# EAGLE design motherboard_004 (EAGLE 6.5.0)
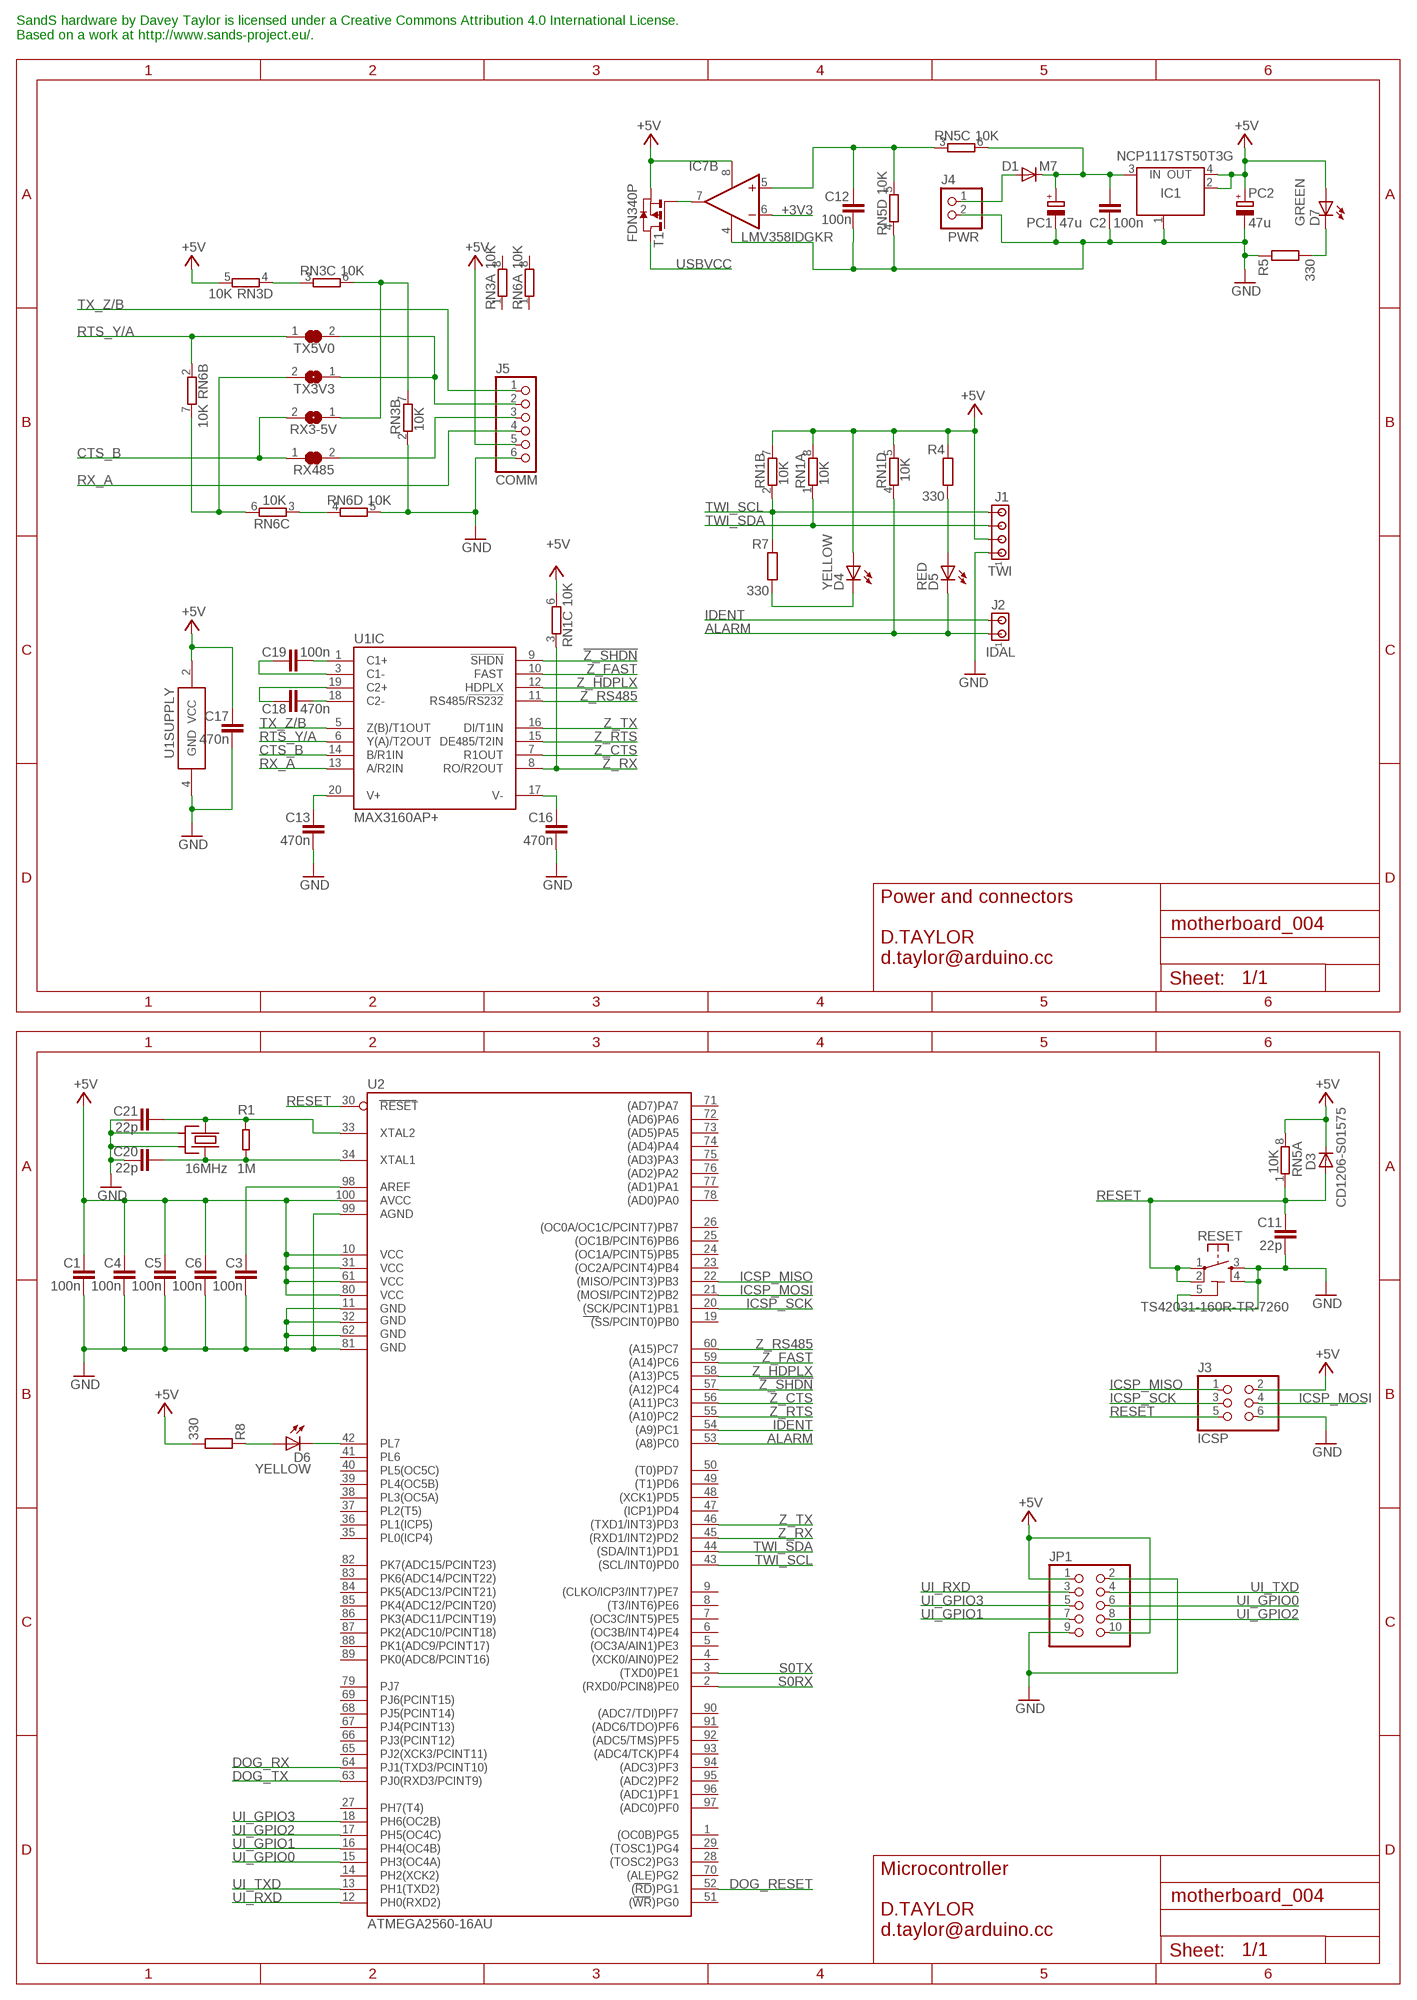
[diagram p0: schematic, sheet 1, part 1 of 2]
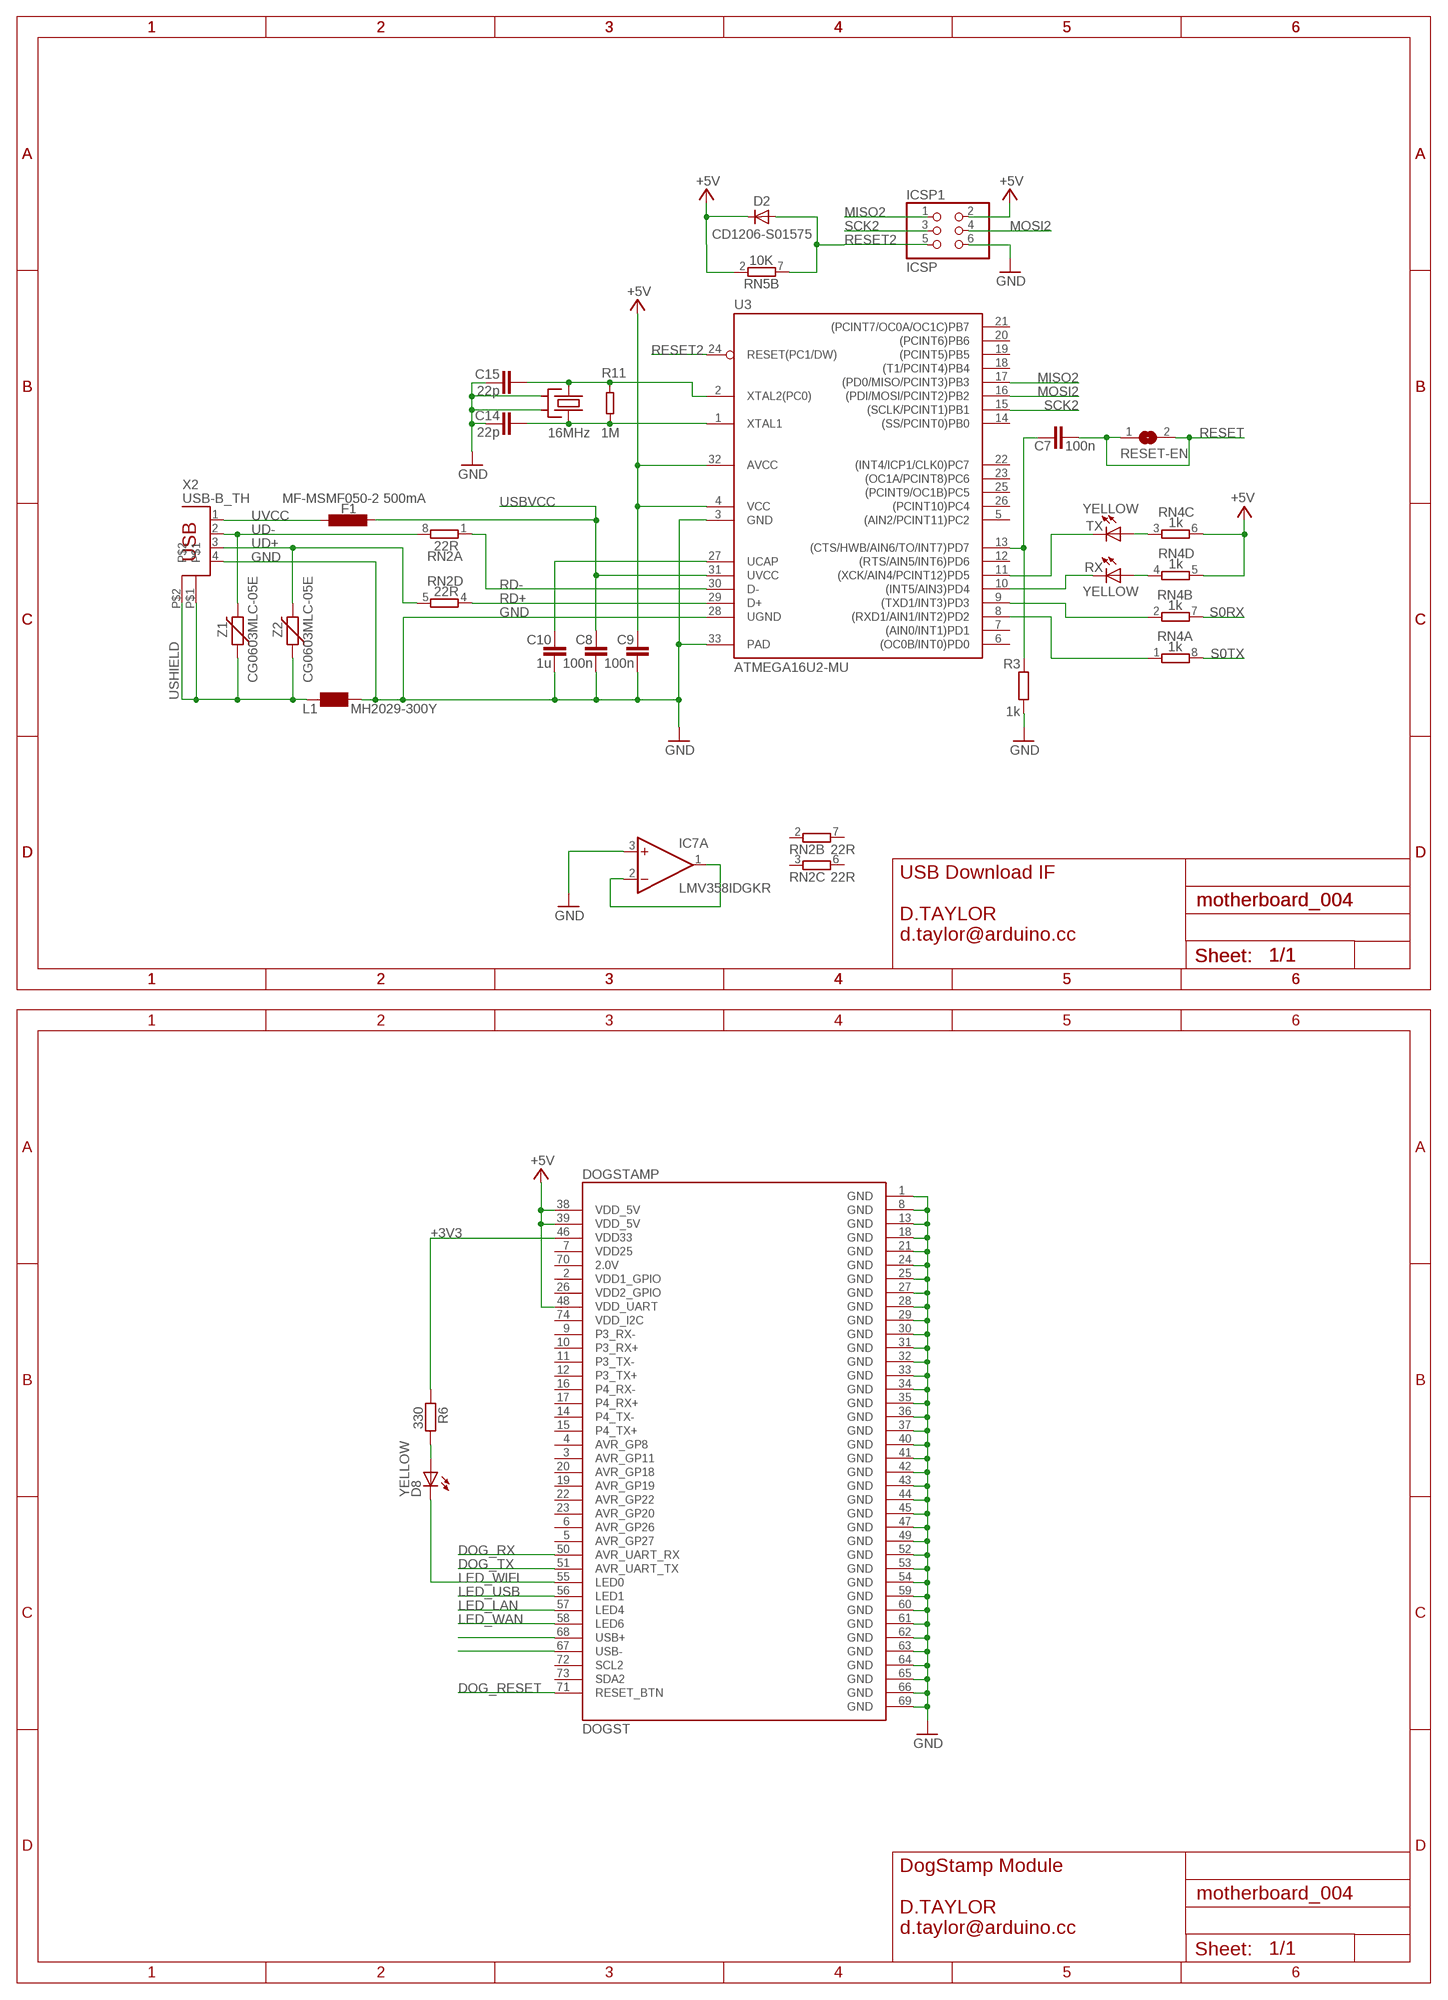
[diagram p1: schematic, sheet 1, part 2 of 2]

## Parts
C1  100n  C-EU0603-RND  [C0603-ROUND]
C2  100n  C-EU0603-RND  [C0603-ROUND]
C3  100n  C-EU0603-RND  [C0603-ROUND]
C4  100n  C-EU0603-RND  [C0603-ROUND]
C5  100n  C-EU0603-RND  [C0603-ROUND]
C6  100n  C-EU0603-RND  [C0603-ROUND]
C7  100n  C-EU0603-RND  [C0603-ROUND]
C8  100n  C-EU0603-RND  [C0603-ROUND]
C9  100n  C-EU0603-RND  [C0603-ROUND]
C10  1u  C-EU0603-RND  [C0603-ROUND]
C11  22p  C-EU0603-RND  [C0603-ROUND]
C12  100n  C-EU0603-RND  [C0603-ROUND]
C13  470n  C-EU0603-RND  [C0603-ROUND]
C14  22p  C-EU0603-RND  [C0603-ROUND]
C15  22p  C-EU0603-RND  [C0603-ROUND]
C16  470n  C-EU0603-RND  [C0603-ROUND]
C17  470n  C-EU0603-RND  [C0603-ROUND]
C18  470n  C-EU0603-RND  [C0603-ROUND]
C19  100n  C-EU0603-RND  [C0603-ROUND]
C20  22p  C-EU0603-RND  [C0603-ROUND]
C21  22p  C-EU0603-RND  [C0603-ROUND]
D1  M7  DIODE-SMB  [SMB]
D2  CD1206-S01575  DIODE-MINIMELF  [MINIMELF]
D3  CD1206-S01575  DIODE-MINIMELF  [MINIMELF]
D4  YELLOW  LEDCHIP-LED0805  [CHIP-LED0805]
D5  RED  LEDCHIP-LED0805  [CHIP-LED0805]
D6  YELLOW  LEDCHIP-LED0805  [CHIP-LED0805]
D7  GREEN  LEDCHIP-LED0805  [CHIP-LED0805]
D8  YELLOW  LEDCHIP-LED0805  [CHIP-LED0805]
DOGSTAMP  DOGST  [DOGST]
F1  MF-MSMF050-2 500mA  L-EUL1812  [L1812]
IC1  NCP1117ST50T3G  MC33269ST-3.3T3  [SOT223]
IC7  LMV358IDGKR  LMV358MMX  [MSOP08]
ICSP1  ICSP  PINHD-2X3  [2X03]
J1  TWI  MTA04-100  [10X04MTA]
J2  IDAL  MTA02-100  [10X02MTA]
J3  ICSP  PINHD-2X3  [2X03]
J4  PWR  MKDS_1,5/2-5,08  [MKDS1,5/2-5,08]
J5  COMM  PINHD-1X6  [1X06]
JP1  PINHD-2X5  [2X05]
L1  MH2029-300Y  WE-CBF_0805  [0805]
PC1  47u  CPOL-EUD  [PANASONIC_D]
PC2  47u  CPOL-EUD  [PANASONIC_D]
R1  1M  R-EU_0603-RND  [R0603-ROUND]
R3  1k  R-EU_R0603  [R0603-ROUND]
R4  330  R-EU_R0603  [R0603-ROUND]
R5  330  R-EU_R0603  [R0603-ROUND]
R6  330  R-EU_R0603  [R0603-ROUND]
R7  330  R-EU_R0603  [R0603-ROUND]
R8  330  R-EU_R0603  [R0603-ROUND]
R11  1M  R-EU_0603-RND  [R0603-ROUND]
RESET  TS42031-160R-TR-7260  TS42  [TS42]
RESET-EN  SJ  [SJ]
RN1  10K  4R-NCAT16  [CAT16]
RN2  22R  4R-NCAY16  [CAY16]
RN3  10K  4R-NCAT16  [CAT16]
RN4  1k  4R-NCAY16  [CAY16]
RN5  10K  4R-NCAT16  [CAT16]
RN6  10K  4R-NCAT16  [CAT16]
RX  YELLOW  LEDCHIP-LED0805  [CHIP-LED0805]
RX3-5V  SJ-NO  [SJ]
RX485  SJ-NC  [SJ-NC]
T1  FDN340P  PMOSSOT23  [SOT-23]
TX  YELLOW  LEDCHIP-LED0805  [CHIP-LED0805]
TX3V3  SJ-NO  [SJ]
TX5V0  SJ-NC  [SJ-NC]
U1  MAX3160AP+  [SSOP20]
U2  ATMEGA2560-16AU  ATMEGA25602560-16AU  [TQFP100]
U3  ATMEGA16U2-MU  [MLF32]
X1  16MHz  CRYSTAL2-KX7  [XTAL-3.2-2.5]
X2  USB-B_TH  PN61729  [PN61729]
X3  16MHz  CRYSTAL2-KX7  [XTAL-3.2-2.5]
Z1  CG0603MLC-05E  VARISTORCN0603  [CT/CN0603]
Z2  CG0603MLC-05E  VARISTORCN0603  [CT/CN0603]

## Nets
!Z_SHDN!: U1.9(IC:!SHDN!) U2.57((A12)PC4)
+3V3 [power]: DOGSTAMP.46(VDD33) IC7.6(B:-IN) R6.2
+5V: C1.1 C4.1 C5.1 C6.1 C9.1 C17.1 D2.C D3.C D4.A D7.A DOGSTAMP.38(VDD_5V) DOGSTAMP.39(VDD_5V) DOGSTAMP.48(VDD_UART) IC1.2(OUT) IC1.4(OUT) IC7.8(P:V+) ICSP1.2 J1.2 J3.2 J5.5 JP1.1 JP1.10 PC2.+ R4.2 R8.1 RN1.5 RN1.6 RN1.7 RN1.8 RN3.5 RN4.5 RN4.6 RN5.2 RN5.8 T1.2(S) U1.2(SUPPLY:VCC) U2.10(VCC) U2.31(VCC1) U2.61(VCC2) U2.80(VCC3) U2.100(AVCC) U3.4(VCC) U3.32(AVCC)
ALARM: D5.C J2.1 RN1.4 U2.53((A8)PC0)
CMP: C12.2 IC7.5(B:+IN) RN5.3 RN5.5
CTS_B: RX3-5V.2 RX485.1 U1.14(IC:B/R1IN)
DOG_RESET: DOGSTAMP.71(RESET_BTN) U2.52((RD)PG1)
DOG_RX: DOGSTAMP.50(AVR_UART_RX) U2.64(PJ1(TXD3/PCINT10))
DOG_TX: DOGSTAMP.51(AVR_UART_TX) U2.63(PJ0(RXD3/PCINT9))
DTR: C7.1 R3.2 U3.13((CTS/HWB/AIN6/TO/INT7)PD7)
GATE_CMD: IC7.7(B:OUT) T1.3(G)
GND: C1.2 C2.2 C3.2 C4.2 C5.2 C6.2 C8.2 C9.2 C10.2 C11.2 C12.1 C13.2 C14.2 C15.2 C16.2 C17.2 C20.2 C21.2 DOGSTAMP.1(GND) DOGSTAMP.8(GND) DOGSTAMP.13(GND) DOGSTAMP.18(GND) DOGSTAMP.21(GND) DOGSTAMP.24(GND) DOGSTAMP.25(GND) DOGSTAMP.27(GND) DOGSTAMP.28(GND) DOGSTAMP.29(GND) DOGSTAMP.30(GND) DOGSTAMP.31(GND) DOGSTAMP.32(GND) DOGSTAMP.33(GND) DOGSTAMP.34(GND) DOGSTAMP.35(GND) DOGSTAMP.36(GND) DOGSTAMP.37(GND) DOGSTAMP.40(GND) DOGSTAMP.41(GND) DOGSTAMP.42(GND) DOGSTAMP.43(GND) DOGSTAMP.44(GND) DOGSTAMP.45(GND) DOGSTAMP.47(GND) DOGSTAMP.49(GND) DOGSTAMP.52(GND) DOGSTAMP.53(GND) DOGSTAMP.54(GND) DOGSTAMP.59(GND) DOGSTAMP.60(GND) DOGSTAMP.61(GND) DOGSTAMP.62(GND) DOGSTAMP.63(GND) DOGSTAMP.64(GND) DOGSTAMP.65(GND) DOGSTAMP.66(GND) DOGSTAMP.69(GND) IC1.1(GND/ADJ) IC7.3(A:+IN) IC7.4(P:V-) ICSP1.6 J1.1 J3.6 J4.2 J5.6 JP1.2 JP1.9 L1.1 PC1.- PC2.- R3.1 R5.2 RESET.3 RESET.4 RESET.5(5-GND) RN3.2 RN5.4 RN6.5 U1.4(SUPPLY:GND) U2.11(GND) U2.32(GND1) U2.62(GND2) U2.81(GND3) U2.99(AGND) U3.3(GND) U3.28(UGND) U3.33(PAD) X1.2(SH1) X1.4(SH2) X2.4 X3.2(SH1) X3.4(SH2)
ICSP_MISO: J3.1 U2.22((MISO/PCINT3)PB3)
ICSP_MOSI: J3.4 U2.21((MOSI/PCINT2)PB2)
ICSP_SCK: J3.3 U2.20((SCK/PCINT1)PB1)
IDENT: J2.2 U2.54((A9)PC1)
LED_LAN: DOGSTAMP.57(LED4)
LED_USB: DOGSTAMP.56(LED1)
LED_WAN: DOGSTAMP.58(LED6)
LED_WIFI: D8.C DOGSTAMP.55(LED0)
M8RXD: RN4.2 U3.9((TXD1/INT3)PD3)
M8TXD: RN4.1 U3.8((RXD1/AIN1/INT2)PD2)
MISO2: ICSP1.1 U3.17((PD0/MISO/PCINT3)PB3)
MOSI2: ICSP1.4 U3.16((PDI/MOSI/PCINT2)PB2)
N$1: C3.1 U2.98(AREF)
N$2: IC7.1(A:OUT) IC7.2(A:-IN)
N$3: C14.1 R11.1 U3.1(XTAL1) X1.3(X2)
N$4: DOGSTAMP.68(USB+)
N$5: D5.A R4.1
N$6: C19.2 U1.1(IC:C1+)
N$7: C18.2 U1.18(IC:C2-)
N$8: C18.1 U1.19(IC:C2+)
N$9: C19.1 U1.3(IC:C1-)
N$10: C13.1 U1.20(IC:V+)
N$11: C16.1 U1.17(IC:V-)
N$12: D7.C R5.1
N$13: D8.A R6.1
N$14: D4.C R7.1
N$15: D6.C U2.42(PL7)
N$16: D6.A R8.2
N$17: DOGSTAMP.67(USB-)
N$18: RN3.3 RN3.4
N$19 [power]: RN3.6 RN3.7 RX3-5V.1
N$20: J5.3 RX485.2
N$21: C20.1 R1.1 U2.34(XTAL1) X3.3(X2)
N$22: J5.2 TX3V3.1 TX5V0.2
N$23: RN6.6 RN6.7 TX3V3.2
N$24: RN6.3 RN6.4
N$54: RN4.4 RX.A
N$55: RN4.3 TX.A
PWRIN [power]: D1.A J4.1
RD+: RN2.4 U3.29(D+)
RD-: RN2.1 U3.30(D-)
RESET: C7.2 C11.1 D3.A J3.5 RESET-EN.1 RESET-EN.2 RESET.1 RESET.2 RN5.1 U2.30(RESET)
RESET2: D2.A ICSP1.5 RN5.7 U3.24(RESET(PC1/DW))
RTS_Y/A: RN6.2 TX5V0.1 U1.6(IC:Y(A)/T2OUT)
RX_A: J5.4 U1.13(IC:A/R2IN)
RXL: RX.C U3.10((INT5/AIN3)PD4)
S0RX: RN4.7 U2.2((RXD0/PCIN8)PE0)
S0TX: RN4.8 U2.3((TXD0)PE1)
SCK2: ICSP1.3 U3.15((SCLK/PCINT1)PB1)
TWI_SCL: J1.4 R7.2 RN1.2 U2.43((SCL/INT0)PD0)
TWI_SDA: J1.3 RN1.1 U2.44((SDA/INT1)PD1)
TX_Z/B: J5.1 U1.5(IC:Z(B)/T1OUT)
TXL: TX.C U3.11((XCK/AIN4/PCINT12)PD5)
UD+: RN2.5 X2.3 Z2.2
UD-: RN2.8 X2.2 Z1.2
UI_GPIO0: JP1.6 U2.15(PH3(OC4A))
UI_GPIO1: JP1.7 U2.16(PH4(OC4B))
UI_GPIO2: JP1.8 U2.17(PH5(OC4C))
UI_GPIO3: JP1.5 U2.18(PH6(OC2B))
UI_RXD: JP1.3 U2.12(PH0(RXD2))
UI_TXD: JP1.4 U2.13(PH1(TXD2))
USBVCC [power usb]: C8.1 F1.1 T1.1(D) U3.31(UVCC)
USHIELD [gnd]: L1.2 X2.P$1 X2.P$2 Z1.1 Z2.1
UVCC [power usb]: F1.2 X2.1
VIN [power]: C2.1 D1.C IC1.3(IN) PC1.+ RN5.6
VUCAP: C10.1 U3.27(UCAP)
XT1: C21.1 R1.2 U2.33(XTAL2) X3.1(X1)
XT2: C15.1 R11.2 U3.2(XTAL2(PC0)) X1.1(X1)
Z_CTS: U1.7(IC:R1OUT) U2.56((A11)PC3)
Z_FAST: U1.10(IC:FAST) U2.59((A14)PC6)
Z_HDPLX: U1.12(IC:HDPLX) U2.58((A13)PC5)
Z_RS485: U1.11(IC:RS485/!RS232!) U2.60((A15)PC7)
Z_RTS: U1.15(IC:DE485/T2IN) U2.55((A10)PC2)
Z_RX: RN1.3 U1.8(IC:RO/R2OUT) U2.45((RXD1/INT2)PD2)
Z_TX: U1.16(IC:DI/T1IN) U2.46((TXD1/INT3)PD3)
Unconnected: DOGSTAMP.2(VDD1_GPIO) DOGSTAMP.3(AVR_GP11) DOGSTAMP.4(AVR_GP8) DOGSTAMP.5(AVR_GP27) DOGSTAMP.6(AVR_GP26) DOGSTAMP.7(VDD25) DOGSTAMP.9(P3_RX-) DOGSTAMP.10(P3_RX+) DOGSTAMP.11(P3_TX-) DOGSTAMP.12(P3_TX+) DOGSTAMP.14(P4_TX-) DOGSTAMP.15(P4_TX+) DOGSTAMP.16(P4_RX-) DOGSTAMP.17(P4_RX+) DOGSTAMP.19(AVR_GP19) DOGSTAMP.20(AVR_GP18) DOGSTAMP.22(AVR_GP22) DOGSTAMP.23(AVR_GP20) DOGSTAMP.26(VDD2_GPIO) DOGSTAMP.70(2.0V) DOGSTAMP.72(SCL2) DOGSTAMP.73(SDA2) DOGSTAMP.74(VDD_I2C) RN2.2 RN2.3 RN2.6 RN2.7 RN3.1 RN3.8 RN6.1 RN6.8 U2.1((OC0B)PG5) U2.4((XCK0/AIN0)PE2) U2.5((OC3A/AIN1)PE3) U2.6((OC3B/INT4)PE4) U2.7((OC3C/INT5)PE5) U2.8((T3/INT6)PE6) U2.9((CLKO/ICP3/INT7)PE7) U2.14(PH2(XCK2)) U2.19((SS/PCINT0)PB0) U2.23((OC2A/PCINT4)PB4) U2.24((OC1A/PCINT5)PB5) U2.25((OC1B/PCINT6)PB6) U2.26((OC0A/OC1C/PCINT7)PB7) U2.27(PH7(T4)) U2.28((TOSC2)PG3) U2.29((TOSC1)PG4) U2.35(PL0(ICP4)) U2.36(PL1(ICP5)) U2.37(PL2(T5)) U2.38(PL3(OC5A)) U2.39(PL4(OC5B)) U2.40(PL5(OC5C)) U2.41(PL6) U2.47((ICP1)PD4) U2.48((XCK1)PD5) U2.49((T1)PD6) U2.50((T0)PD7) U2.51((WR)PG0) U2.65(PJ2(XCK3/PCINT11)) U2.66(PJ3(PCINT12)) U2.67(PJ4(PCINT13)) U2.68(PJ5(PCINT14)) U2.69(PJ6(PCINT15)) U2.70((ALE)PG2) U2.71((AD7)PA7) U2.72((AD6)PA6) U2.73((AD5)PA5) U2.74((AD4)PA4) U2.75((AD3)PA3) U2.76((AD2)PA2) U2.77((AD1)PA1) U2.78((AD0)PA0) U2.79(PJ7) U2.82(PK7(ADC15/PCINT23)) U2.83(PK6(ADC14/PCINT22)) U2.84(PK5(ADC13/PCINT21)) U2.85(PK4(ADC12/PCINT20)) U2.86(PK3(ADC11/PCINT19)) U2.87(PK2(ADC10/PCINT18)) U2.88(PK1(ADC9/PCINT17)) U2.89(PK0(ADC8/PCINT16)) U2.90((ADC7/TDI)PF7) U2.91((ADC6/TDO)PF6) U2.92((ADC5/TMS)PF5) U2.93((ADC4/TCK)PF4) U2.94((ADC3)PF3) U2.95((ADC2)PF2) U2.96((ADC1)PF1) U2.97((ADC0)PF0) U3.5((AIN2/PCINT11)PC2) U3.6((OC0B/INT0)PD0) U3.7((AIN0/INT1)PD1) U3.12((RTS/AIN5/INT6)PD6) U3.14((SS/PCINT0)PB0) U3.18((T1/PCINT4)PB4) U3.19((PCINT5)PB5) U3.20((PCINT6)PB6) U3.21((PCINT7/OC0A/OC1C)PB7) U3.22((INT4/ICP1/CLK0)PC7) U3.23((OC1A/PCINT8)PC6) U3.25((PCINT9/OC1B)PC5) U3.26((PCINT10)PC4)

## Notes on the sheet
- SandS hardware by Davey Taylor is licensed under a Creative Commons Attribution 4.0 International License.
  Based on a work at http://www.sands-project.eu/.
- Power and connectors
  
  D.TAYLOR
  d.taylor@arduino.cc
- USB Download IF
  
  D.TAYLOR
  d.taylor@arduino.cc
- Microcontroller
  
  D.TAYLOR
  d.taylor@arduino.cc
- DogStamp Module
  
  D.TAYLOR
  d.taylor@arduino.cc

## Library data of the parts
C1-C21 = SmartPrj:C-EU: CAPACITOR, European symbol
D1-D3 = diode:DIODE-: DIODE
D4-D8 RX TX = led:LED: LED
DOGSTAMP = d_taylor:DOGST
F1 = rcl:L-EU: INDUCTOR, European symbol
IC1 = linear:MC33269ST*: Adjustable Output Low Dropout Voltage Regulator 800 mA Source: http://www.onsemi.com/pub/Collateral/MC33269-D.PDF
IC7 = linear:LMV358?*: Dual General Purpose, Low Voltage, Rail-to-Rail Output Operational Amplifiers Source: http://www.national.com/mpf/LM/LMV321.html http://www.national.com/dt/lmv_qual.pdf
ICSP1 = SmartPrj:PINHD-2X3: PIN HEADER
J1 = con-amp:MTA04-100: AMP connector
J2 = con-amp:MTA02-100: AMP connector
J3 = pinhead:PINHD-2X3: PIN HEADER
J4 = d_taylor:MKDS_1,5/2-5,08: Screw terminal header
J5 = pinhead:PINHD-1X6: PIN HEADER
JP1 = pinhead:PINHD-2X5: PIN HEADER
L1 = wuerth-elektronik:WE-CBF: SMD EMI Suppression Ferrite Beads
PC1 PC2 = rcl:CPOL-EU: POLARIZED CAPACITOR, European symbol
R1 R11 = d_taylor:R-EU_: RESISTOR, European symbol
R3-R8 = SmartPrj:R-EU_: RESISTOR, European symbol
RESET = SmartPrj:TS42: TS42 Dongnan Electronics Tact switch VDC 12V - 50mA
RESET-EN = jumper:SJ: SMD solder JUMPER
RN1-RN6 = resistor-dil:4R-N: Array Chip Resistor Source: RS Component / Phycomp; OC_FARNELL: unknown; OC_NEWARK: unknown
RX3-5V TX3V3 = d_taylor:SJ?-NO: SMD solder JUMPER
RX485 TX5V0 = d_taylor:SJ?-NC
T1 = zetex:PMOSSOT23: MOS FET; OC_FARNELL: unknown; OC_NEWARK: unknown
U1 = d_taylor:MAX3160*AP+
U2 = SmartPrj:ATMEGA2560: MICROCONTROLLER 64/128/256 Kbytes FLASH 4 Kbytes EEPROM 8 Kbytes SRAM 86 General Purpose I/O pins 12-channels16-bit PWM 4 x Serial USARTs 16-channels 10-bit A/D
U3 = SmartPrj:ATMEGA16U2-
X1 X3 = d_taylor:CRYSTAL2: KX7 SMD crystal
X2 = SmartPrj:PN61729: BERG USB connector
Z1 Z2 = varistor:VARISTOR: VARISTOR

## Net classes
0 default: width 0.254 mm, drill 0.406 mm, clearance 0.178 mm
1 power: width 0.254 mm, drill 0.406 mm, clearance 0.178 mm
2 gnd: width 0.254 mm, drill 0.406 mm, clearance 0.178 mm
3 power usb: width 0.254 mm, drill 0.406 mm, clearance 0.178 mm

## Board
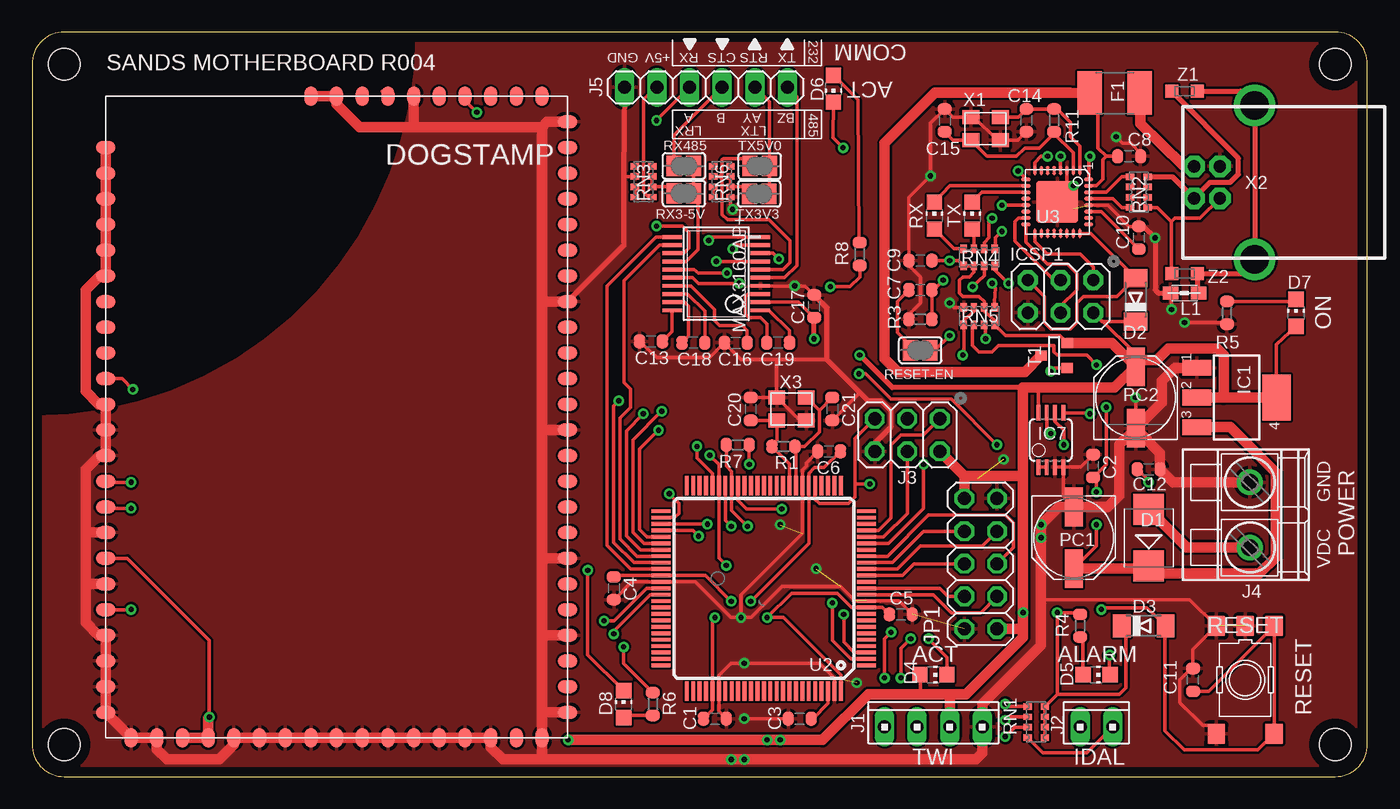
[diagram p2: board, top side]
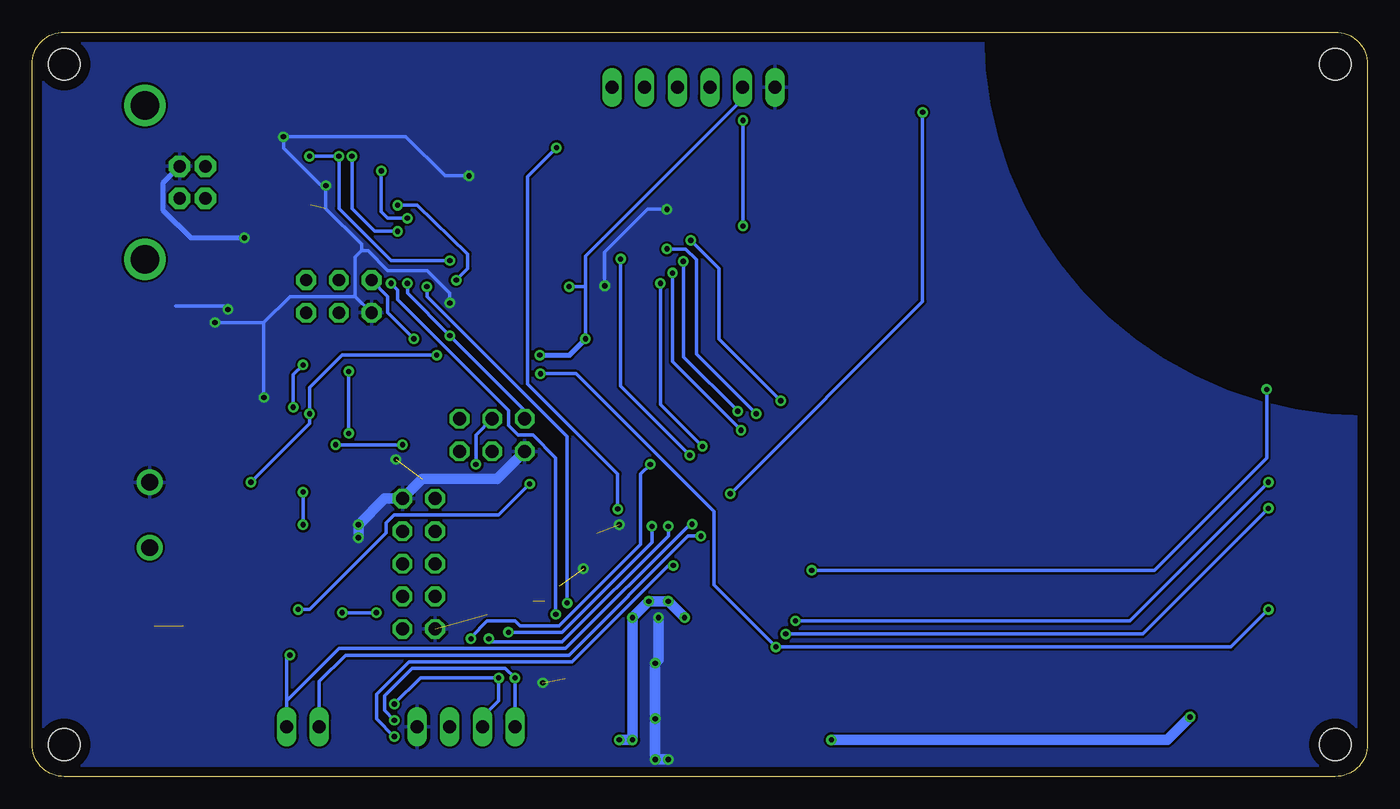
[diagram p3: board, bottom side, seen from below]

Size 104 x 58 mm. Coordinates in mm from the lower left corner, seen from the top.
Outline: 2.5,0 101.5,0 arc90 104,2.5 104,55.5 arc90 101.5,58 2.5,58 arc90 0,55.5 0,2.5 arc90 2.5,0
Copper layers (1*16): Top 0.035mm / dielectric 1.5mm / Bottom 0.035mm
Design rules "default *": minimum track width 10mil, minimum drill 16mil, track to track 7mil, track to pad 7mil, pad to pad 7mil, via to via 7mil, smd to smd 7mil, copper to edge 30mil, drill to drill 8mil, minimum pad ring 10mil, minimum via ring 8mil, stop-mask expansion 4mil, vias tented up to drill 0mil, thermal gap 10mil
Holes 2.5 mm at 2.5,2.5 2.5,55.5 101.5,2.5 101.5,55.5

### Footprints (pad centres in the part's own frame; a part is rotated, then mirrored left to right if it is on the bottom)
C0603-ROUND = smd 0.898 x 1.1: 1 -0.889,0; 2 0.889,0
SMB = smd 2.4 x 2.4: A 2.2,0; C -2.2,0
MINIMELF = smd 1.4 x 1.8: A 1.7,0; C -1.7,0
CHIP-LED0805 = smd 1.2 x 1.2: A 0,-1.05; C 0,1.05
DOGST = smd 1 x 1.5: 1 -23,18; 2 -21,18; 3 -19,18; 4 -17,18; 5 -15,18; 6 -13,18; 7 -11,18; 8 -9,18; 9 -7,18; 10 -5,18; 11 -3,18; 12 -1,18; 13 1,18; 14 3,18; 15 5,18; 16 7,18; 17 9,18; 18 11,18; 19 13,18; 20 15,18; 21 17,18; 22 19,18; 23 21,18; 24 23,18; 42 23,-18; 43 21,-18; 44 19,-18; 45 17,-18; 46 15,-18; 47 13,-18; 48 11,-18; 49 9,-18; 50 7,-18; 51 5,-18; 52 3,-18; 53 1,-18; 54 -1,-18; 55 -3,-18; 56 -5,-18; 57 -7,-18; 58 -9,-18; 59 -11,-18; 60 -13,-18; 61 -15,-18; 62 -17,-18; 63 -19,-18; 64 -21,-18 | smd 1.5 x 1: 25 25,16; 26 25,14; 27 25,12; 28 25,10; 29 25,8; 30 25,6; 31 25,4; 32 25,2; 33 25,0; 34 25,-2; 35 25,-4; 36 25,-6; 37 25,-8; 38 25,-10; 39 25,-12; 40 25,-14; 41 25,-16; 65 -25,-2; 66 -25,0; 67 -25,2; 68 -25,4; 69 -25,6; 70 -25,8; 71 -25,10; 72 -25,12; 73 -25,14; 74 -25,16
L1812 = smd 1.9 x 3.4: 1 -1.95,0; 2 1.95,0
SOT223 = smd 1.219 x 2.235: 1 -2.311,-3.099; 2 0,-3.099; 3 2.311,-3.099 | smd 3.6 x 2.2: 4 0,3.099
MSOP08 = smd 0.3 x 1.2: 1 -0.976,-2.113; 2 -0.326,-2.113; 3 0.324,-2.113; 4 0.974,-2.113; 5 0.974,2.112; 6 0.324,2.112; 7 -0.326,2.112; 8 -0.976,2.112
2X03 = drill 0.95 pad 1.55 octagon: 1 -2.54,-1.27; 2 -2.54,1.27; 3 0,-1.27; 4 0,1.27; 5 2.54,-1.27; 6 2.54,1.27
10X04MTA = drill 1.016 long: 1 3.81,0; 2 1.27,0; 3 -1.27,0; 4 -3.81,0
10X02MTA = drill 1.016 long: 1 1.27,0; 2 -1.27,0
2X03' = drill 1.016 octagon: 1 -2.54,-1.27; 2 -2.54,1.27; 3 0,-1.27; 4 0,1.27; 5 2.54,-1.27; 6 2.54,1.27
MKDS1,5/2-5,08 = drill 1.3 pad 2: 1 -2.54,0; 2 2.54,0
1X06 = drill 1.016 long: 1 -6.35,0; 2 -3.81,0; 3 -1.27,0; 4 1.27,0; 5 3.81,0; 6 6.35,0
2X05 = drill 1.016 octagon: 1 -5.08,-1.27; 2 -5.08,1.27; 3 -2.54,-1.27; 4 -2.54,1.27; 5 0,-1.27; 6 0,1.27; 7 2.54,-1.27; 8 2.54,1.27; 9 5.08,-1.27; 10 5.08,1.27
0805 = smd 1.2 x 1: 1 -1.1,0; 2 1.1,0
PANASONIC_D = smd 3 x 1.4: + 2.4,0; - -2.4,0
R0603-ROUND = smd 0.898 x 1.1: 1 -0.889,0; 2 0.889,0
TS42 = smd 1.6 x 1.4: 1 -4.2,2.25; 2 4.2,2.25; 3 -4.2,-2.25; 4 4.2,-2.25; 5 -4.2,0
SJ = smd 1.168 x 1.6: 1 -0.762,0; 2 0.762,0
CAT16 = smd 0.5 x 0.65: 1 -1.2,-0.675; 2 -0.4,-0.675; 3 0.4,-0.675; 4 1.2,-0.675; 5 1.2,0.675; 6 0.4,0.675; 7 -0.4,0.675; 8 -1.2,0.675
CAY16 = smd 0.5 x 0.65: 1 -1.2,-0.675; 2 -0.4,-0.675; 3 0.4,-0.675; 4 1.2,-0.675; 5 1.2,0.675; 6 0.4,0.675; 7 -0.4,0.675; 8 -1.2,0.675
SJ-NC = smd 1.168 x 1.6: 1 -0.762,0; 2 0.762,0
SOT-23 = smd 0.787 x 0.889: 1 0.025,-1.016; 2 -0.94,1.016; 3 0.991,1.016
SSOP20 = smd 0.305 x 1.5: 1 -2.857,-3.43; 2 -2.222,-3.43; 3 -1.587,-3.43; 4 -0.952,-3.43; 5 -0.317,-3.43; 6 0.318,-3.43; 7 0.953,-3.43; 8 1.588,-3.43; 9 2.223,-3.43; 10 2.858,-3.43; 11 2.858,3.43; 12 2.223,3.43; 13 1.588,3.43; 14 0.953,3.43; 15 0.318,3.43; 16 -0.317,3.43; 17 -0.952,3.43; 18 -1.587,3.43; 19 -2.222,3.43; 20 -2.857,3.43
TQFP100 = smd 1.5 x 0.3: 1 -8,6; 2 -8,5.5; 3 -8,5; 4 -8,4.5; 5 -8,4; 6 -8,3.5; 7 -8,3; 8 -8,2.5; 9 -8,2; 10 -8,1.5; 11 -8,1; 12 -8,0.5; 13 -8,0; 14 -8,-0.5; 15 -8,-1; 16 -8,-1.5; 17 -8,-2; 18 -8,-2.5; 19 -8,-3; 20 -8,-3.5; 21 -8,-4; 22 -8,-4.5; 23 -8,-5; 24 -8,-5.5; 25 -8,-6; 51 8,-6; 52 8,-5.5; 53 8,-5; 54 8,-4.5; 55 8,-4; 56 8,-3.5; 57 8,-3; 58 8,-2.5; 59 8,-2; 60 8,-1.5; 61 8,-1; 62 8,-0.5; 63 8,0; 64 8,0.5; 65 8,1; 66 8,1.5; 67 8,2; 68 8,2.5; 69 8,3; 70 8,3.5; 71 8,4; 72 8,4.5; 73 8,5; 74 8,5.5; 75 8,6 | smd 0.3 x 1.5: 26 -6,-8; 27 -5.5,-8; 28 -5,-8; 29 -4.5,-8; 30 -4,-8; 31 -3.5,-8; 32 -3,-8; 33 -2.5,-8; 34 -2,-8; 35 -1.5,-8; 36 -1,-8; 37 -0.5,-8; 38 0,-8; 39 0.5,-8; 40 1,-8; 41 1.5,-8; 42 2,-8; 43 2.5,-8; 44 3,-8; 45 3.5,-8; 46 4,-8; 47 4.5,-8; 48 5,-8; 49 5.5,-8; 50 6,-8; 76 6,8; 77 5.5,8; 78 5,8; 79 4.5,8; 80 4,8; 81 3.5,8; 82 3,8; 83 2.5,8; 84 2,8; 85 1.5,8; 86 1,8; 87 0.5,8; 88 0,8; 89 -0.5,8; 90 -1,8; 91 -1.5,8; 92 -2,8; 93 -2.5,8; 94 -3,8; 95 -3.5,8; 96 -4,8; 97 -4.5,8; 98 -5,8; 99 -5.5,8; 100 -6,8
MLF32 = smd 0.7 x 0.28: 1 -2.45,1.75; 2 -2.45,1.25; 3 -2.45,0.75; 4 -2.45,0.25; 5 -2.45,-0.25; 6 -2.45,-0.75; 7 -2.45,-1.25; 8 -2.45,-1.75; 17 2.45,-1.75; 18 2.45,-1.25; 19 2.45,-0.75; 20 2.45,-0.25; 21 2.45,0.25; 22 2.45,0.75; 23 2.45,1.25; 24 2.45,1.75 | smd 0.28 x 0.7: 9 -1.75,-2.45; 10 -1.25,-2.45; 11 -0.75,-2.45; 12 -0.25,-2.45; 13 0.25,-2.45; 14 0.75,-2.45; 15 1.25,-2.45; 16 1.75,-2.45; 25 1.75,2.45; 26 1.25,2.45; 27 0.75,2.45; 28 0.25,2.45; 29 -0.25,2.45; 30 -0.75,2.45; 31 -1.25,2.45; 32 -1.75,2.45 | smd 3.254 x 3.254: 33 0,0
XTAL-3.2-2.5 = smd 1.3 x 1.1: 1 -1.15,-0.9; 2 1.15,-0.9; 3 1.15,0.9; 4 -1.15,0.9
PN61729 = drill 0.95 pad 1.676 octagon: 1 1.25,4.71; 2 -1.25,4.71; 3 -1.25,2.71; 4 1.25,2.71 | drill 2.2: P$1 -6,0; P$2 6,0
CT/CN0603 = smd 1 x 1: 1 -1,0; 2 1,0

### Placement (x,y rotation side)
C1  53.18,4.51 0 top
C2  82.64,24.2 90 top
C3  59.78,4.51 180 top
C4  45.31,14.67 270 top
C5  67.66,12.64 0 top
C6  62.07,25.34 180 top
C7  69.18,37.91 180 top
C8  85.44,48.33 0 top
C9  69.18,40.2 180 top
C10  86.2,41.98 90 top
C11  90.42,7.53 90 top
C12  86.96,23.94 180 top
C13  48.2,33.9 180 top
C14  77.44,51.12 270 top
C15  71.09,51.12 90 top
C16  54.81,33.8 180 top
C17  60.9,36.64 90 top
C18  51.5,33.8 0 top
C19  58.11,33.8 0 top
C20  55.98,28.64 90 top
C21  62.33,28.64 270 top
D1  86.96,18.61 90 top
D2  85.95,37.15 90 top
D3  86.58,11.75 0 top
D4  70.2,7.94 270 top
D5  82.9,7.94 270 top
D6  62.42,53.59 180 top
D7  98.44,36.13 0 top
D8  46.07,5.65 0 top
DOGSTAMP  23.72,28.01 270 top
F1  84.32,53.25 0 top
IC1  93.82,29.53 270 top
IC7  79.34,26.23 0 top
ICSP1  80.11,37.4 180 top
J1  70.2,3.88 0 top
J2  82.9,3.88 0 top
J3  ICSP  [2X03']  68.17,26.61 180 top
J4  94.84,20.39 90 top
J5  52.48,53.7 180 top
JP1  73.88,16.58 90 top
L1  89.76,37.66 0 top
PC1  81.12,18.61 270 top
PC2  85.95,29.53 90 top
R1  58.52,25.72 0 top
R3  69.18,35.63 0 top
R4  81.63,11.75 90 top
R5  93.06,36.13 270 top
R6  48.35,5.65 90 top
R7  54.96,25.85 180 top
R8  64.46,40.71 90 top
R11  79.6,51.12 270 top
RESET  94.48,7.53 270 top
RESET-EN  69.18,33.21 0 top
RN1  78.2,4.26 270 top
RN2  86.2,45.53 270 top
RN3  47.62,46.34 270 top
RN4  73.75,40.45 180 top
RN5  73.75,35.88 180 top
RN6  53.71,46.34 270 top
RX  70.28,43.7 0 top
RX3-5V  50.77,45.43 0 top
RX485  50.77,47.56 180 top
T1  79.6,32.83 270 top
TX  73.22,43.7 0 top
TX3V3  56.62,45.4 180 top
TX5V0  56.66,47.56 0 top
U1  53.28,39.18 90 top
U2  56.99,14.67 180 top
U3  79.85,44.77 270 top
X1  74.26,50.48 0 top
X2  95.22,46.29 90 top
X3  59.15,28.64 180 top
Z1  89.76,53.41 180 top
Z2  89.76,39.18 180 top

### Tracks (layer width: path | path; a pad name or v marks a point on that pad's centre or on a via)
!Z_SHDN!  (via drill 0.41)
  Top 0.254: v47.59,28.26 46.3,26.94 46.3,18.76 47.39,17.67 U2.57 | U1.9 54.84,41.41 v54.55,41.11
  Bottom 0.254: v54.55,41.11 53.1,41.11 52.27,40.27 52.27,32.91 48.53,29.17 v47.59,28.26
+3V3  (via drill 0.41)
  Top 0.254: DOGSTAMP.46 7.7,13.01 v7.71,13.02 | v80.36,25.85 80.36,26.99 79.67,27.68 IC7.6 | R6.2 46.07,8.83 v46.07,10.1 | v64.41,31.38 64.92,31.38 66.9,29.4 71.6,29.4 v75.15,25.85
  Bottom 0.254: v7.71,13.02 10.64,10.1 v46.07,10.1 50.9,14.93 50.9,20.64 61.64,31.38 v64.41,31.38 | v75.15,25.85 v80.36,25.85
+5V  (via drill 0.41)
  Top 0.254: v80.11,48.33 U3.4 | U3.32 82.3,48.49 v82.39,48.33 | C9.1 v71.47,40.2 72.13,40.2 RN4.5 RN4.6 73.36,39.29 72.99,38.93 72.48,38.93 72.23,38.67 72.23,37.66 72.48,37.4 73.75,37.4 74.16,37 RN5.2 74.16,36.24 74.14,36.26 74.95,35.57 RN5.8 | PC2.+ 86.45,32.44 ICSP1.2 83.33,35.45 D2.C | RN5.8 74.85,35.06 | IC7.8 78.37,30.08 78.58,30.29 | T1.2 80.03,34.36 75.8,34.36 RN5.8 | 78.88,5.44 RN1.7 RN1.6 RN1.5 | C17.1 59.7,36.96 U1.2 | RN1.8 78.88,5.44 | 78.88,5.44 79.85,6.42 | 79.85,6.42 84.68,6.42 85.19,6.92 85.19,11.37 85.06,11.5 D3.C | 79.85,6.42 v79.85,12.77 81.5,12.77 R4.2 | v53.18,12.38 52.99,12.2 U2.80 52.99,5.21 C1.1 | v54.45,13.65 52.44,15.67 U2.61 45.7,15.67 C4.1 | v55.98,13.65 60.49,18.17 U2.31 60.49,23.63 60.93,24.07 61.69,24.07 C6.1 | U2.100 62.99,7.91 58.52,12.38 v57.24,12.38 59.15,14.29 62.71,14.29 63.83,13.17 U2.10 66.24,13.17 C5.1 | D7.A 96.92,33.66 IC1.4 | D4.A 69.18,7.91 69.18,6.42 | R8.1 64.46,38.93 63.7,38.17 v62.17,38.17 | DOGSTAMP.48 7.41,17.01 13.81,10.61 v13.81,4.64 | RN3.5 48.01,45.15 47.62,45.53 47.62,52.77 J5.5
  Top 0.406: 77.18,30.29 67,30.29 v64.46,32.83 | v60.9,34.1 C17.1
  Top 0.813: IC1.4 92.81,29.53 | 92.81,29.53 IC1.2 | 86.45,32.44 87.58,32.44 88.49,33.34 92.3,33.34 92.81,32.83 92.81,29.53 | T1.2 84.11,33.77 PC2.+ 84.31,30.29 78.58,30.29 77.18,30.29 77.18,23.43 | 77.18,23.43 v77.18,12.77 77.18,11.62 | 77.18,11.62 77.18,10.86 72.74,6.42 71.47,6.42 | 71.47,6.42 J1.2 71.47,3.37 | 71.47,6.42 69.18,6.42 65.12,6.42 61.56,2.86 v58.26,2.86 v57.24,2.86 v41.75,2.86 | v13.81,4.64 13.72,4.54 DOGSTAMP.38 DOGSTAMP.39 | JP1.10 72.61,23.43 | 72.61,23.43 J3.2 | 72.61,23.43 77.18,23.43 | JP1.1 76.93,11.5 77.18,11.62
  Bottom 0.254: v82.39,48.33 v80.11,48.33 80.11,44.26 76.04,40.2 v71.47,40.2 | v77.18,12.77 v79.85,12.77 | v60.9,34.1 60.9,38.17 | v62.17,38.17 60.9,38.17 | 60.9,38.17 60.9,40.55 48.67,52.79 J5.5
  Bottom 0.406: v64.46,32.83 62.12,32.83 v60.9,34.1
  Bottom 0.813: v41.75,2.86 15.59,2.86 v13.81,4.64 | v58.26,2.86 v57.24,2.86 v57.24,12.38 v55.98,13.65 v54.45,13.65 v53.18,12.38
ALARM  (via drill 0.41)
  Top 0.254: v52.59,19.67 U2.53 | RN1.4 78.74,1.84 82.14,1.84 J2.1 | D5.C 83.92,7.97 v83.92,9.46
  Bottom 0.254: J2.1 84.17,5.91 | 84.17,5.91 80.11,9.97 62.45,9.97 52.8,19.62 v52.59,19.67 | v83.92,9.46 84.17,9.21 84.17,5.91
CMP  (via drill 0.41)
  Top 0.254: C12.2 86.96,23.05 v86.96,22.93 | v82.39,28.26 82.31,28.34 IC7.5 | RN5.3 73.36,36.24 73.37,36.26 72.56,35.57 RN5.5 72.56,32.76 v72.48,32.83
  Bottom 0.254: v86.96,22.93 82.39,27.5 v82.39,28.26 82.39,30.29 79.85,32.83 v72.48,32.83
CTS_B
  Top 0.254: U1.14 50.93,40.13 51.86,41.06 51.86,44.69 RX3-5V.2 RX485.1
DOG_RESET  (via drill 0.41)
  Top 0.254: U2.52 50.05,20.17 50.39,20.51 50.39,21.27 v49.62,22.04 | v34.64,51.76 34,52.39 33.75,52.78 DOGSTAMP.71
  Bottom 0.254: v49.62,22.04 34.64,37.02 v34.64,51.76
DOG_RX  (via drill 0.41)
  Top 0.254: U2.64 48.11,14.17 45.31,11.37 v45.31,11.12 | v7.71,20.89 5.83,20.89 DOGSTAMP.50
  Bottom 0.254: v45.31,11.12 17.49,11.12 v7.71,20.89
DOG_TX  (via drill 0.41)
  Top 0.254: U2.63 47.85,14.67 45.31,12.13 v44.55,12.13 | v7.71,22.93 5.8,22.93 DOGSTAMP.51
  Bottom 0.254: v44.55,12.13 18.51,12.13 v7.71,22.93
DTR  (via drill 0.41)
  Top 0.254: U3.13 v75.54,44.52 v75.53,44.52 | v70.96,38.67 70.2,37.91 C7.1 R3.2
  Bottom 0.254: v70.96,38.67 70.07,39.56 70.07,40.71 74.01,44.52 v75.53,44.52
GATE_CMD  (via drill 0.41)
  Top 0.254: v79.34,31.56 79.62,31.84 T1.3 | IC7.7 79.02,27.06 v79.34,26.74
  Bottom 0.254: v79.34,26.74 v79.34,31.56
GND  (via drill 0.41)  (8 unrouted)
  Top 0.254: U3.3 80.6,45.52 U3.33 80.61,44.77 v81.12,46.04 | C8.2 86.33,48.58 85.57,49.34 84.93,49.34 v84.42,49.85 | IC1.1 91.51,31.84 91.53,31.82 | v85.95,29.53 PC2.- | IC7.4 81.67,24.11 C2.2 | IC7.4 80.32,21.81 PC1.- | IC7.3 IC7.4 | R3.1 68.29,36.01 69.18,36.9 69.18,38.93 68.29,39.82 C9.2 68.29,45.13 v69.97,46.8 69.97,50.89 C15.2 71.71,51.38 X1.4 73.36,51.38 75.16,49.59 X1.2 | 60.71,37.72 C17.2 60.2,38.23 v59.4,38.23 U1.4 | C13.2 48.69,32.63 52.75,32.63 C16.2 53.92,33.77 55.21,32.48 57.98,32.48 | RESET.4 91.59,3.98 91.18,3.98 89.4,5.76 89.4,7.53 90.29,8.42 C11.2 90.42,9.92 RESET.3 90.18,13.78 78.58,13.78 | C3.2 v55.47,4.51 | v55.21,12.38 55.98,12.38 58.39,14.8 62.96,14.8 64.09,13.67 67.52,13.67 C5.2 | v55.21,12.38 55.21,14.16 59.99,18.94 U2.32 59.99,23.89 60.29,24.2 60.29,24.45 C6.2 | v55.21,12.38 54.45,12.38 51.66,15.17 U2.62 46.7,15.17 C4.2 | U2.99 62.49,7.65 61.31,8.83 v55.47,8.83 54.45,8.83 53.49,7.87 U2.81 53.49,5.09 C1.2 | R5.2 92.93,35.37 v89.76,35.37 | RN5.4 71.81,36.55 v71.47,36.9 | 75.42,49.6 X1.2 | C14.2 76.79,49.59 X1.2 | C21.2 64.48,29.91 | X3.4 59.8,27.74 X3.2 | C20.2 57.99,29.53 X3.2 | X3.2 58.02,29.54 | U3.28 83.78,44.52 85.44,42.87 C10.2 | v88.74,36.39 88.74,37.66 L1.1 | 57.98,32.48 61.92,32.48 | X3.2 57.98,29.56 57.98,32.48 | RN3.2 46.08,46.74 46.07,46.95 | RN6.5 54.39,44.37 v54.56,44.2
  Top 0.406: C17.2 61.92,36.52 61.92,32.48 64.48,29.91 65.12,29.28 66.14,29.28 66.9,28.51 66.9,27.24 65.63,25.97 J3.6 | J5.6 46.07,46.95 46.07,41.36 DOGSTAMP.8 | C10.2 86.58,42.87 v87.47,41.98 87.47,37.91 87.72,37.66 L1.1
  Top 0.813: J4.2 88.87,22.93 C12.1 87.85,25.23 PC2.- | IC1.1 89.02,31.84 87.98,30.8 87.98,29.16 PC2.- | PC2.- 84.68,25.86 84.68,21.91 83.78,21.01 PC1.- 79.97,21.01 v78.58,19.62 v78.58,18.61 78.58,13.78 78.58,10.23 74.01,5.65 J1.1 74.01,1.84 73.5,1.34 v55.47,1.34 v54.45,1.34 39.72,1.34 | 4.16,15.01 4.16,19.01 | DOGSTAMP.64 DOGSTAMP.63 DOGSTAMP.62 DOGSTAMP.61 DOGSTAMP.60 DOGSTAMP.59 5.25,39.01 4.16,37.91 4.16,30.04 5.19,29.01 DOGSTAMP.54 DOGSTAMP.53 DOGSTAMP.52 5.67,24.96 5.17,24.96 4.16,23.94 4.16,19.01 | DOGSTAMP.49 4.16,19.01 | DOGSTAMP.47 4.16,15.01 | DOGSTAMP.41 | 39.72,1.34 DOGSTAMP.25 39.72,5.01 | 39.72,5.01 39.72,11.01 | 39.72,11.01 39.72,17.01 | 39.72,17.01 39.72,27.01 | 39.72,27.01 39.72,37.01 | 39.72,37.01 39.72,50.61 | 39.72,50.61 29.72,50.61 | 29.72,50.61 25.5,50.61 23.72,52.39 DOGSTAMP.66 DOGSTAMP.65 | DOGSTAMP.69 29.72,50.61 | DOGSTAMP.1 40.1,51.01 39.72,50.61 | DOGSTAMP.8 39.72,37.01 | DOGSTAMP.18 39.72,17.01 | DOGSTAMP.13 39.72,27.01 | DOGSTAMP.24 39.72,5.01 | DOGSTAMP.21 39.72,11.01 | 39.72,1.34 36.67,1.34 35.72,2.29 DOGSTAMP.27 DOGSTAMP.28 DOGSTAMP.29 DOGSTAMP.30 DOGSTAMP.31 DOGSTAMP.32 DOGSTAMP.33 DOGSTAMP.34 DOGSTAMP.35 DOGSTAMP.36 DOGSTAMP.37 15.72,2.48 14.57,1.34 10.51,1.34 9.72,2.13 DOGSTAMP.40 DOGSTAMP.41 | DOGSTAMP.41 DOGSTAMP.42 DOGSTAMP.43 DOGSTAMP.44 DOGSTAMP.45 5.16,11.01 4.16,12 4.16,15.01
  Bottom 0.254: ICSP1.6 78.83,37.4 | 78.83,37.4 78.83,40.45 78.33,40.96 | v89.76,35.37 85.95,35.37 | 85.95,35.37 83.92,37.4 78.83,37.4 | 85.95,35.37 v85.95,29.53 | v71.47,36.9 71.47,37.66 73.25,39.44 76.3,39.44 77.82,40.96 78.33,40.96 | 78.33,40.96 78.33,41.47 81.12,44.26 v81.12,46.04 81.5,46.04 84.42,48.96 v84.42,49.85 74.9,49.85 71.85,46.8 v69.97,46.8 | 92.81,36.64 89,36.64 v88.74,36.39 | v59.4,38.23 59.4,40.86 56.05,44.21 56.04,44.2 v54.56,44.2
  Bottom 0.406: X2.4 93.82,46.23 93.82,44.13 91.66,41.98 v87.47,41.98
  Bottom 0.813: v54.45,1.34 v55.47,1.34 v55.47,4.51 v55.47,8.83 55.21,9.08 v55.21,12.38 | v78.58,18.61 v78.58,19.62 76.55,21.66 JP1.9 73.63,23.18 67.79,23.18 J3.6
  other vias: 61.05,16.2 58.26,19.62 75.66,24.7 64.23,7.3
  pour Bottom: 0.2,28 0.2,0.2 103.8,0.2 103.8,57.8 30,57.8 arc-90
  pour Top: 0.2,28 0.2,0.2 103.8,0.2 103.8,57.8 30,57.8 arc-90
ICSP_MISO
  Top 0.254: U2.22 65.94,19.17 66.9,20.13 66.9,25.85 67.66,26.61 69.44,26.61 J3.1
ICSP_MOSI
  Top 0.254: U2.21 66.33,18.67 68.17,20.51 J3.4
ICSP_SCK  (via drill 0.41)
  Top 0.254: U2.20 66.71,18.17 69.44,20.89 v69.44,24.32
  Bottom 0.254: v69.44,24.32 69.44,26.61 J3.3
IDENT  (via drill 0.41)
  Top 0.254: v51.91,18.73 51.48,19.17 U2.54
  Bottom 0.254: J2.2 81.63,7.43 79.6,9.46 62.2,9.46 52.93,18.73 v51.91,18.73
LED_WIFI  (via drill 0.41)
  Top 0.254: D8.C 43.27,9.5 v43.27,16.07 | v7.84,30.16 7,31.01 DOGSTAMP.55
  Bottom 0.254: v43.27,16.07 16.61,16.07 7.84,24.83 v7.84,30.16
M8RXD  (via drill 0.41)
  Top 0.254: U3.9 77.4,46.59 v76.8,47.18 | v74.77,43.5 74.52,43.25 74.52,41.98 74.16,41.61 RN4.2
  Bottom 0.254: v76.8,47.18 76.8,44.01 76.3,43.5 v74.77,43.5
M8TXD  (via drill 0.41)
  Top 0.254: RN4.1 75.04,41.21 75.04,41.99 v75.53,42.48 | U3.8 78.1,47.85 78.58,48.33 v79.09,48.33
  Bottom 0.254: v79.09,48.33 79.09,44.26 77.31,42.48 v75.53,42.48
MISO2
  Top 0.254: U3.17 78.1,41.69 79.09,40.71 81.63,40.71 82.64,39.69 ICSP1.1
MOSI2
  Top 0.254: U3.16 77.4,41.63 79.09,39.94 80.61,39.94 81.38,39.18 81.38,37.91 80.11,36.64 ICSP1.4
N$1
  Top 0.254: C3.1 60.8,4.51 61.99,5.7 U2.98
N$2
  Top 0.254: IC7.2 IC7.1
N$3
  Top 0.254: U3.1 81.6,49.12 80.87,49.85 80.87,50.99 79.85,52.01 R11.1 C14.1 76.81,51.38 X1.3 75.42,51.37
N$4
  Top 0.254: 27.27,53.41 27.44,53.41 DOGSTAMP.68
N$5
  Top 0.254: R4.1 81.85,10.64 D5.A
N$6
  Top 0.254: U1.1 57.41,36.33 59,34.74 C19.2
N$7
  Top 0.254: U1.18 51.06,37.59 52.39,36.26 C18.2
N$8
  Top 0.254: U1.19 50.81,36.96 51.12,36.64 51.12,34.3 C18.1
N$9
  Top 0.254: U1.3 55.76,37.59 55.57,37.4 55.57,36.01 55.82,35.75 56.71,35.75 57.22,35.24 C19.1
N$10
  Top 0.254: C13.1 49.85,34.66 U1.20
N$11
  Top 0.254: U1.17 51.31,38.23 53.16,36.39 53.16,35.52 53.54,35.14 55.31,35.14 55.7,34.76 C16.1
N$12
  Top 0.254: D7.C 98.38,37.02 R5.1
N$13
  Top 0.254: D8.A 46.23,4.76 R6.1
N$14  (via drill 0.41)
  Top 0.254: D4.C 71.25,9.3 v69.82,10.73 | v55.85,24.32 R7.1
  Bottom 0.254: v69.82,10.73 69.82,10.86 68.55,12.13 66.39,12.13 66.01,11.75 62.96,11.75 56.61,18.1 56.61,23.56 v55.85,24.32
N$15  (via drill 0.41)
  Top 0.254: U2.42 54.99,21.5 55.65,20.84 v58.39,20.84 | D6.C 62.39,49.76 v63.16,48.99
  Bottom 0.254: v58.39,20.84 58.39,23.59 65.4,30.6 65.4,46.75 v63.16,48.99
N$16
  Top 0.254: D6.A 64.31,52.73 64.39,41.66 R8.2
N$18
  Top 0.254: RN3.4 RN3.3
N$19
  Top 0.254: RN3.7 RN3.6 49.49,45.95 RX3-5V.1
N$20
  Top 0.254: RX485.2 50.01,49.95 J5.3
N$21
  Top 0.254: U2.34 58.99,24.36 R1.1 58,26.09 X3.3 C20.1
N$22
  Top 0.254: TX3V3.1 57.42,45.44 TX5V0.2 57.42,52.56 J5.2
N$23
  Top 0.254: RN6.7 RN6.6 55.32,45.95 TX3V3.2
N$24
  Top 0.254: RN6.3 RN6.4
N$54
  Top 0.254: RX.A 71.8,41.13 RN4.4
N$55
  Top 0.254: RN4.3 73.36,43.07 TX.A
PWRIN
  Top 0.813: J4.1 89.92,17.85 D1.A
RD+
  Top 0.254: RN2.4 84.86,44.33 84.17,45.02 U3.29
RD-
  Top 0.254: RN2.1 84.86,46.73 83.65,45.52 U3.30
RESET  (via drill 0.41)
  Top 0.254: RN5.1 74.95,36.97 75.03,38.04 v74.77,38.42 | C7.2 67.41,37.02 67.41,34.61 68.42,33.59 RESET-EN.1 RESET-EN.2 70.33,33.21 v71.47,34.36 | C11.1 91.64,6.64 RESET.1 RESET.2 95.45,2.07 89.73,2.07 88.23,3.57 88.23,11.75 D3.A 86.84,13.15 83.41,13.15 v83.28,13.02 | U2.30 60.99,21.59 61.31,21.27 63.59,21.27 64.1,21.78 64.1,22.8 | 64.1,22.8 64.1,26.36 J3.5 | v65.25,22.8 64.1,22.8
  Bottom 0.254: v74.77,38.42 74.77,37.66 v71.47,34.36 65.63,28.51 J3.5 | v83.28,13.02 82.39,13.02 76.42,18.99 76.42,19.75 75.79,20.39 67.66,20.39 v65.25,22.8
RESET2  (via drill 0.41)
  Top 0.254: U3.24 82.48,42.32 D2.A 84.5,37.4 81.88,37.4 81.38,36.9 81.38,35.37 80.87,34.86 79.34,34.86 78.83,35.37 78.83,37.4 ICSP1.5 | RN5.7 74.26,35.1 v74.26,34.1
  Bottom 0.254: v74.26,34.1 76.3,36.13 76.3,37.4 ICSP1.5
RTS_Y/A
  Top 0.254: RN6.2 53.55,46.74 | 53.55,46.74 53.75,46.94 53.75,48.06 53.85,48.16 55.47,48.16 55.47,47.99 TX5V0.1 | U1.6 58.5,39.5 59.03,40.03 59.03,41.76 57.4,43.38 54.15,43.38 53.75,43.79 53.75,46.53 53.55,46.73 53.55,46.74
RX_A  (via drill 0.41)
  Top 0.254: U1.13 50.78,40.77 51.17,41.16 51.17,42.38 50.67,42.89 v48.63,42.89 | v48.63,51.12 J5.4
  Bottom 0.254: v48.63,42.89 v48.63,51.12
RXL
  Top 0.254: U3.10 71.49,46.02 RX.C
S0RX  (via drill 0.41)
  Top 0.254: RN4.7 74.16,39.04 v73.25,38.17 | U2.2 63.76,9.17 62.33,10.61 v62.33,13.53
  Bottom 0.254: v73.25,38.17 73.25,37.4 62.33,26.48 v62.33,13.53
S0TX  (via drill 0.41)
  Top 0.254: RN4.8 74.95,39.51 v76.04,38.42 | v63.21,12.64 63.21,10.48 64.02,9.67 U2.3
  Bottom 0.254: v76.04,38.42 75.53,37.91 75.53,37.15 66.9,28.51 66.9,27.37 66.14,26.61 64.99,26.61 63.21,24.83 v63.21,12.64
SCK2
  Top 0.254: U3.15 76.82,43.52 76.55,43.25 76.55,41.72 79.6,38.67 ICSP1.3
TWI_SCL  (via drill 0.41)
  Top 0.254: v75.79,4.38 76.06,4.66 RN1.2 | v66.39,7.69 66.39,10.73 v66.9,11.24 | v55.72,19.5 54.49,20.73 U2.43 54.49,23.77 54.07,24.2 R7.2
  Bottom 0.254: J1.4 v66.39,7.69 67.15,8.45 74.39,8.45 76.55,6.29 76.55,5.15 v75.79,4.38 | v66.9,11.24 62.71,11.24 55.72,18.23 v55.72,19.5
TWI_SDA  (via drill 0.41)
  Top 0.254: RN1.1 75.98,5.46 v75.79,5.65 | v67.66,7.69 67.66,9.97 v68.42,10.73 | v54.45,19.5 53.99,19.96 U2.44
  Bottom 0.254: J1.3 68.93,4.64 67.66,5.91 v67.66,7.69 73.75,7.69 v75.79,5.65 | v68.42,10.73 68.17,10.48 62.71,10.48 54.45,18.73 v54.45,19.5
TX_Z/B
  Top 0.254: U1.5 58.6,38.87 59.56,39.82 59.56,52.98 J5.1
TXL
  Top 0.254: U3.11 73.96,45.52 TX.C
UD+
  Top 0.254: RN2.5 87.66,44.33 88.74,43.25 | 88.74,43.25 89,43.5 90.96,43.5 X2.3 | 88.74,43.25 88.74,39.2 Z2.2
UD-
  Top 0.406: Z1.2 88.76,53.39 93.95,48.17 93.95,46.93 93.31,46.29 91.76,46.29 X2.2 88.82,46.73 RN2.8
UI_GPIO0
  Top 0.254: U2.15 67.77,15.67 68.67,16.58 JP1.6
UI_GPIO1
  Top 0.254: U2.16 67.38,16.17 69.18,17.97 74.01,17.97 JP1.7
UI_GPIO2
  Top 0.254: U2.17 66.99,16.67 69.44,19.12 JP1.8
UI_GPIO3
  Top 0.254: JP1.5 76.42,17.85 76.42,19.75 75.79,20.39 69.82,20.39 66.6,17.17 U2.18
UI_RXD
  Top 0.254: U2.12 70.19,14.17 71.6,12.77 73.88,12.77 JP1.3
UI_TXD
  Top 0.254: U2.13 70.71,14.67 71.34,14.04 JP1.4
USBVCC
  Top 0.254: U3.31 82.88,46.02 83.41,46.55 83.41,48.07 83.66,48.33 | F1.1 83.03,51.71 83.03,48.96 83.66,48.33 | C8.1 83.66,48.33
  Top 0.813: F1.1 80.82,53.28 70.33,53.28 66.39,49.34 66.39,32.58 67.43,31.54 77.31,31.54 T1.1
USHIELD
  Top 0.406: Z1.1 94.11,53.41 X2.P$2 X2.P$1 94.23,39.18 Z2.1 90.76,37.88 L1.2
UVCC
  Top 0.813: X2.1 89.62,47.62 86.33,50.87 86.27,52.99 F1.2
VIN  (via drill 0.41)
  Top 0.254: v82.9,22.16 82.9,23.05 C2.1 83.66,24.32 v83.66,28.77 | PC1.+ 82.9,17.99 v82.9,19.62 | RN5.6 73.25,35.1 73.25,33.59 73.75,33.09 74.77,33.09 75.28,33.59 79.6,33.59 79.6,33.09 79.85,32.83 82.14,32.83 v82.9,32.07
  Top 0.813: PC1.+ 86.76,16.21 D1.C 87.56,15.81 95.6,15.81 96.87,17.08 96.87,23.69 93.34,27.22 IC1.3
  Bottom 0.254: v82.9,22.16 v82.9,19.62 | v83.66,28.77 83.66,31.31 v82.9,32.07
VUCAP
  Top 0.254: U3.27 83.27,44.02 C10.1
XT1
  Top 0.254: 60.04,29.8 X3.1 61.31,28.53 | U2.33 59.49,25.63 R1.2 60.17,25.72 61.31,26.86 61.31,28.53 | C21.1 62.31,29.53 61.31,28.53
XT2
  Top 0.254: U3.2 81.1,48.6 79.6,50.1 | C15.1 71.73,49.59 X1.1 74.37,48.33 76.68,48.33 77.31,48.96 78.45,48.96 79.6,50.1 | 79.6,50.1 R11.2
Z_CTS  (via drill 0.41)
  Top 0.254: v49.04,28.46 46.81,26.23 46.81,19.01 47.65,18.17 U2.56 | U1.7 53.47,40.13 v53.28,40.15
  Bottom 0.254: v53.28,40.15 53.28,32.7 v49.04,28.46
Z_FAST  (via drill 0.41)
  Top 0.254: v45.69,29.28 45.28,28.87 45.28,18.25 46.86,16.67 U2.59 | U1.10 52.97,42.04 v52.7,41.77
  Bottom 0.254: v45.69,29.28 50.49,34.08 50.49,39.56 v52.7,41.77
Z_HDPLX
  Top 0.254: U2.58 47.12,17.17 45.79,18.51 45.79,27.95 46.6,28.77 46.6,30.19 46.09,30.7 46.09,38.62 48.88,41.41 U1.12
Z_RS485
  Top 0.254: U2.60 46.6,16.17 44.77,18 44.77,38.22 48.6,42.04 U1.11
Z_RTS  (via drill 0.41)
  Top 0.254: v48.79,26.99 47.31,25.52 47.31,19.27 47.91,18.67 U2.55 | U1.15 51.57,39.5 51.89,39.23 v54.12,39.23
  Bottom 0.254: v54.12,39.23 54.12,32.32 v48.79,26.99
Z_RX  (via drill 0.41)
  Top 0.254: 52.77,25.01 v52.77,25.03 53.49,24.32 U2.45 53.49,17.03 v54.07,16.45 | RN1.3 76.53,3.86 v75.79,3.11 | U1.8 57.71,40.77 v58.16,40.33
  Bottom 0.254: v75.79,3.11 77.18,4.51 77.18,6.42 74.64,8.96 61.94,8.96 54.45,16.45 v54.07,16.45 | v58.16,40.33 58.16,30.42 v52.77,25.03
Z_TX  (via drill 0.41)
  Top 0.254: v51.78,25.72 51.78,24.81 52.99,23.6 U2.46 | U1.16 51.44,38.87 51.89,38.42 v55.06,38.42
  Bottom 0.254: v55.06,38.42 55.06,29 v51.78,25.72

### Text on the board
tPlace: 232 | COMM | GND | +5V | RX | CTS | RTS | TX | SANDS MOTHERBOARD R004 | ACT | A | B | AY | BZ | 485 | LRX | LTX | ON | GND | POWER | VDC | ACT | ALARM | RESET | TWI | IDAL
